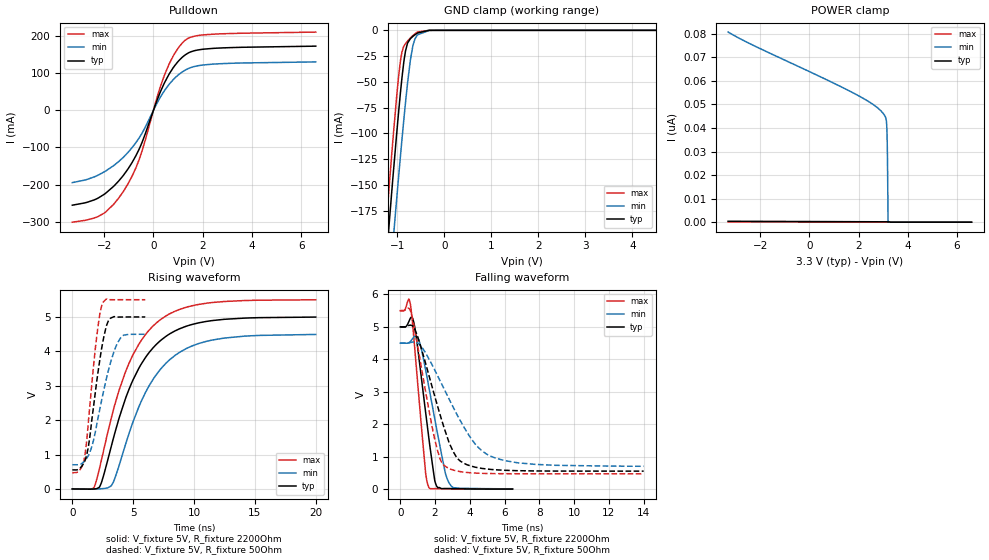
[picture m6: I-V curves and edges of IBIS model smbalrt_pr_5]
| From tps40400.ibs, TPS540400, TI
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|   smbalrt_pr_5 Model
[Model]   smbalrt_pr_5
Model_type   Open_sink
Polarity   Inverting
Vmeas = 1.65
Vref = 3.3
Cref = 2pF
Rref = 2200
|   typ   min   max
|   (nom PVT)   (fast PVT)   (slow PVT)
C_comp   1.150e-12   1.129e-12   1.173e-12
| Where nom  PVT is Nominal Process, 3.3V, 25C
|   Fast PVT is Strong Process,  3.4V, -40C
|   Slow PVT is Weak Process,   3.2V, 125C
[Voltage Range]   3.3   3.2   3.4
|Junction Temperature
[Temperature Range]   25   125   -40
[Pullup Reference]   3.3   3.2   3.4
[Pulldown Reference]   0   0   0
[Power Clamp Reference]   3.3   3.2   3.4
[GND Clamp Reference]   0   0   0
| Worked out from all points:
|   slope of the pulldown table from 0 to 0.495 V, typ, clamps not added: 6.2 ohm
|   GND clamp passes 1 mA (typ) near -0.42 V on its own axis
|   falling waveform, V_fixture 5V, R_fixture 2200Ohm: 20-80 % time 704ps typ, 950ps min, 533ps max; typ from 5 V to 0.012 V
|   rising waveform, V_fixture 5V, R_fixture 2200Ohm: 20-80 % time 3.36ns typ, 3.5ns min, 3.27ns max; typ from 0.012 V to 5 V
|   falling waveform, V_fixture 5V, R_fixture 50Ohm: 20-80 % time 1.47ns typ, 2.29ns min, 1.04ns max; typ from 5 V to 0.564 V
|   rising waveform, V_fixture 5V, R_fixture 50Ohm: 20-80 % time 1.01ns typ, 1.42ns min, 826ps max; typ from 0.564 V to 5 V
[Pulldown]
|   Voltage   I(typ)   I(min)   I(max)
-3.3V     -255.3mA   -194.7mA   -301.1mA
-2.41V    -241.1mA   -179.3mA   -289.8mA
-2.001V   -225.9mA   -165.7mA   -276.5mA
-1.221V   -174.9mA   -126.2mA   -218mA
-861.6mV  -139.6mA   -99.81mA   -175.9mA
-576.8mV  -103.8mA   -73.77mA   -131.6mA
148.5mV   27.58mA    19.62mA    35.46mA
460.4mV   75.5mA     53.98mA    96.63mA
858mV     119.4mA    85.93mA    152.1mA
1.293V    149mA      108mA      188.4mA
2.422V    166.3mA    124mA      204.5mA
6.597V    172.3mA    129.9mA    210.1mA
[GND Clamp]
|   Voltage   I(typ)   I(min)   I(max)
-3.3V     -1.486A    -1.512A    -1.478A
-1.277V   -244.6mA   -306.4mA   -209.5mA
-1.127V   -159.8mA   -223.3mA   -123.2mA
-1.092V   -140.4mA   -204mA     -103.6mA
-1.019V   -101.2mA   -164.7mA   -65.03mA
-940.4mV  -62.25mA   -124.1mA   -30.94mA
-903mV    -45.55mA   -105.3mA   -20.73mA
-828.3mV  -20.01mA   -69.82mA   -12.85mA
-724mV    -8.058mA   -28.57mA   -7.408mA
-672.8mV  -5.897mA   -15.15mA   -5.152mA
-570.4mV  -2.564mA   -4.36mA    -1.648mA
6.597V    0A         0A         0A
[POWER Clamp]
|   Voltage   I(typ)   I(min)   I(max)
-3.3V     396.6pA    80.72nA    94.42pA
1.782V    213.1pA    54.91nA    23.02pA
2.504V    185.7pA    50.61nA    12.87pA
2.998V    163.7pA    46.27nA    5.93pA
3.116V    156.8pA    43.98nA    4.264pA
3.148V    154.5pA    40.78nA    3.813pA
3.161V    153.5pA    36.79nA    3.633pA
3.174V    152.5pA    29.42nA    3.452pA
3.186V    151.4pA    17.72nA    3.272pA
3.199V    150.2pA    1.198nA    3.091pA
3.206V    149.5pA    0A         3.001pA
6.597V    0A         0A         0A
[Ramp]
R_load = 2200
|   typ   min   max
dV/dt_r   2.99122/3.35523e-09   2.68718/3.49898e-09   3.29313/3.26358e-09
dV/dt_f   2.99306/7.01417e-10   2.6911/9.50329e-10   3.29407/5.32252e-10
[Falling Waveform]
V_fixture = 5V
V_fixture_min = 4.5V
V_fixture_max = 5.5V
R_fixture = 2200Ohm
|   Time   V(typ)   V(min)   V(max)
0s        5V         4.5V       5.5V
586ps     5.27V      4.555V     5.689V
786ps     5.123V     4.693V     4.64V
1.072ns   4.061V     4.592V     2.84V
1.466ns   2.347V     3.665V     471.1mV
1.64ns    1.605V     3.164V     69mV
2.088ns   105.4mV    1.88V      25.51mV
2.594ns   31.2mV     500.8mV    18.14mV
2.938ns   27.59mV    101.9mV    15.21mV
6.458ns   12.19mV    18.55mV    9.936mV
|   2e-08   0.0115667   0.0146771   0.00987613
[Rising Waveform]
V_fixture = 5V
V_fixture_min = 4.5V
V_fixture_max = 5.5V
R_fixture = 2200Ohm
|   Time   V(typ)   V(min)   V(max)
0s        11.57mV    14.67mV    9.876mV
1.796ns   11.1mV     8.835mV    61.94mV
2.382ns   184mV      17.12mV    835.3mV
3.204ns   1.251V     103.4mV    2.074V
4.94ns    3.138V     1.911V     3.871V
6.006ns   3.823V     2.806V     4.488V
7.134ns   4.281V     3.436V     4.893V
8.806ns   4.657V     3.973V     5.218V
11.01ns   4.87V      4.292V     5.398V
20ns      4.997V     4.493V     5.498V
[Falling Waveform]
V_fixture = 5V
V_fixture_min = 4.5V
V_fixture_max = 5.5V
R_fixture = 50Ohm
|   Time   V(typ)   V(min)   V(max)
0s        5V         4.5V       5.5V
614ps     5.053V     4.522V     5.455V
986ps     4.724V     4.511V     4.462V
1.912ns   3.006V     3.75V      1.719V
2.268ns   2.342V     3.369V     973.1mV
2.546ns   1.859V     3.065V     727.3mV
3.468ns   867.2mV    2.103V     548.2mV
4.396ns   677.6mV    1.345V     502.9mV
5.46ns    606.5mV    969.3mV    488mV
14ns      564.3mV    713.6mV    482.6mV
[Rising Waveform]
V_fixture = 5V
V_fixture_min = 4.5V
V_fixture_max = 5.5V
R_fixture = 50Ohm
|   Time   V(typ)   V(min)   V(max)
0s        564.3mV    713.5mV    482.6mV
584ps     600mV      717.5mV    552.9mV
978ps     785.4mV    810.6mV    877.1mV
1.326ns   1.255V     985.7mV    1.99V
1.912ns   2.874V     1.701V     4.155V
2.268ns   3.776V     2.338V     5.105V
2.45ns    4.17V      2.658V     5.361V
2.964ns   4.886V     3.448V     5.501V
3.956ns   4.998V     4.389V     5.501V
5.994ns   5V         4.499V     5.5V
